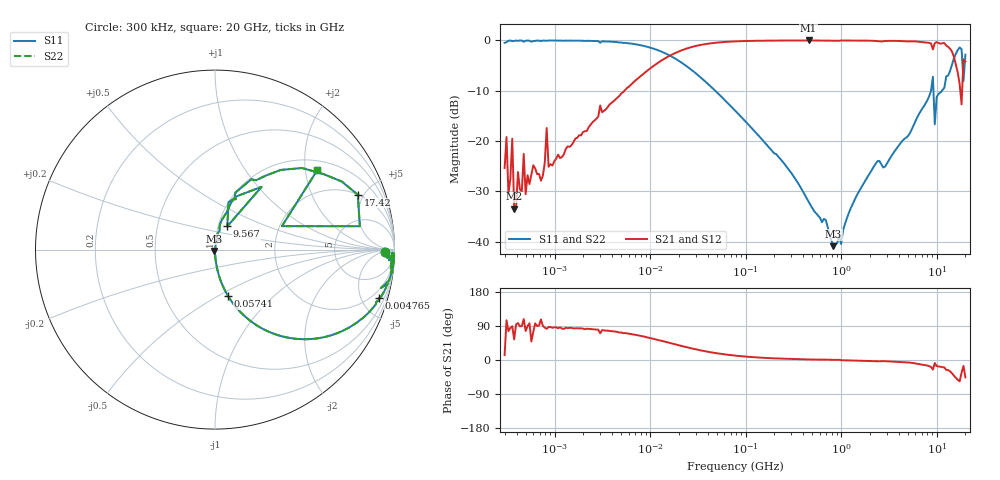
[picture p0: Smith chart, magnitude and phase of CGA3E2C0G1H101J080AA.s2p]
! S-parameter Generated by TDK Corporation
! Copyright(C) 2015 TDK Corporation.
! All Rights Reserved.
! TDK P/N: CGA3E2C0G1H101J080AA (Multilayer Ceramic Chip Capacitors)
! Property: C=100pF
! Size(LxWxT): 1.6x0.8x0.8mm, 0.063x0.031x0.031inches
! Model Type: s2p (Touchstone File Format Version 1.0)
! Frequency: DC=Yes Start=0.3MHz Stop=20000MHz 243points Log-sweep
! Note:
! Model Generated on Jun. 23, 2015
! Hash(MD5):
! Port Assignments:
!  1 ---| |--- 2
! Applicable Conditions:
!  Temperature = 25 degC
!  DC Bias Voltage = 0 V
!  Small Signal Operation
! Terms and conditions regarding TDK Simulation Models
! (1)This simulation model is being provided solely for informational purposes. Please refer to the specifications of the products in terms of detailed characteristics of such products.
! (2)In no event shall TDK Corporation of any of its subsidiaries be liable for any loss or damage arising, directly or indirectly,
!  From any information contained in this simulation model, including, but not limited to loss or damages arising from any inaccuracies, omissions or errors in connection with such information.
! (3)Any and all copyrights on this simulation model are owned by TDK Corporation.
!  Duplication or redistribution of this simulation model without prior written permission from TDK Corporation is prohibited.
! (4)This simulation model is subject to any modification or change without any prior notice.
! (5)Neither TDK Corporation nor any of its subsidiaries shall make any warranty, express or implied,
!  Including but not limited to the correctness, implied warranties of merchantability and fitness for a particular purpose with respect to this simulation models.
! (6)The use of this simulation model shall be deemed to have consented to the terms and conditions hereof.
# MHz S MA R 50
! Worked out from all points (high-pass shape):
!   242 points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, 300 kHz to 20 GHz, reference 50 ohm
!   highest |S21| = 0.00 dB at 456.8 MHz (marker M1); lowest = -33.4 dB at 377.7 kHz (marker M2)
!   |S21| within 3 dB of the highest: 16.19 MHz to 14.99 GHz (14.98 GHz wide, 200 % of centre)
!   lowest |S11| = -40.9 dB at 831.6 MHz (marker M3), VSWR 1.02, Z = 49.6 - j0.788 ohm
!   |S11| at or under -10 dB: 48.19 MHz to 8.732 GHz (8.684 GHz wide, 198 % of centre); 9.263 GHz to 11.36 GHz (2.098 GHz wide, 20.3 % of centre)
!   |S22| runs from -40.9 to 0.0 dB; largest |S21 - S12| = 0
!   S11 on the Smith chart (normalised r, x): 300 kHz: 35, -8; 4.765 MHz: 1.18, -6.78; 57.41 MHz: 1.00, -0.56; 9.567 GHz: 1.11, +0.29; 17.42 GHz: 2.02, +4.52; 20 GHz: 1.26, +2.32
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0.3  0.9473 -0.7  0.05415 13.0  0.05415 13.0  0.9473 -0.7
0.3141503  0.9612 -2.8  0.11 104.9  0.11 104.9  0.9612 -2.8
0.328968  0.9933 -1.7  0.0298 76.1  0.0298 76.1  0.9933 -1.7
0.3607332  0.9848 -6.1  0.1058 89.1  0.1058 89.1  0.9848 -6.1
0.3777482  0.9877 -0.9  0.02128 54.1  0.02128 54.1  0.9877 -0.9
0.4756456  0.9702 -3.5  0.07472 108.0  0.07472 108.0  0.9702 -3.5
0.7201607  0.986 -2.1  0.04052 107.0  0.04052 107.0  0.986 -2.1
0.8269477  0.9909 -7.7  0.1349 82.3  0.1349 82.3  0.9909 -7.7
0.8659529  0.9984 -3.2  0.05564 86.8  0.05564 86.8  0.9984 -3.2
1.985118  0.9924 -7.1  0.1232 82.9  0.1232 82.9  0.9924 -7.1
4.765345  0.9524 -16.3  0.2811 72.2  0.2811 72.2  0.9524 -16.3
12.54397  0.789 -37.9  0.6136 52.1  0.6136 52.1  0.789 -37.9
57.40771  0.269 -74.3  0.9626 15.6  0.9626 15.6  0.269 -74.3
79.26541  0.1972 -78.5  0.9798 11.4  0.9798 11.4  0.1972 -78.5
456.7726  0.02498 -88.6  0.9997 1.4  0.9997 1.4  0.02498 -88.6
500.8786  0.02152 -91.0  0.9989 1.2  0.9989 1.2  0.02152 -91.0
831.5931  0.009059 -118.7  0.9956 0.5  0.9956 0.5  0.009059 -118.7
3165.055  0.06482 80.0  0.9908 -3.7  0.9908 -3.7  0.06482 80.0
9135.962  0.4354 53.4  0.8146 -25.2  0.8146 -25.2  0.4354 53.4
9566.884  0.1469 62.1  0.9406 -8.0  0.9406 -8.0  0.1469 62.1
17417.32  0.8524 21.0  0.3679 -56.2  0.3679 -56.2  0.8524 21.0
20000  0.7213 37.8  0.6172 -45.8  0.6172 -45.8  0.7213 37.8
